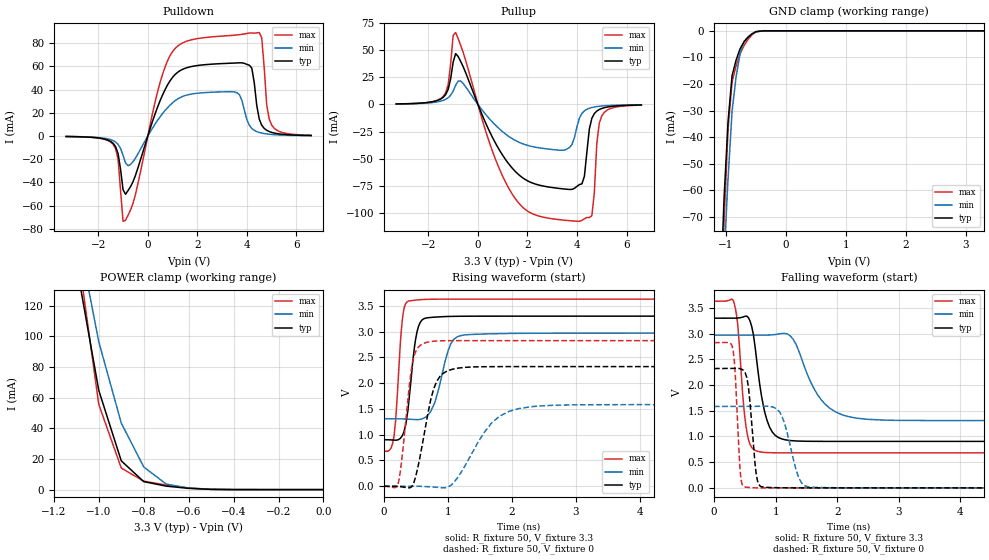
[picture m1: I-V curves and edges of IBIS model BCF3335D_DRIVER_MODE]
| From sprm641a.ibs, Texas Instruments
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|   Model Cell BCF3335D_DRIVER_MODE
|BCF3335D_DRIVER_MODE
[Model]   BCF3335D_DRIVER_MODE
Model_type   I/O
Polarity   Non-Inverting
Enable   Active-Low
Vinl =  0.8
Vinh =  2
Cref =  15.0000pF
Rref =  100.0000M
Vref =  0V
Vmeas =  1.65
C_comp   1.199917p   1.06526p   1.338254p
[Model Spec]
Vinl   0.8   0.8   0.8
Vinh   2   2   2
[Temperature Range]   25   155   -40
[Voltage Range]   3.3   2.97   3.63
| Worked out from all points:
|   slope of the pulldown table from 0 to 0.495 V, typ, clamps not added: 16.3 ohm
|   slope of the pullup table from 0 to 0.495 V, typ, clamps not added: 18.9 ohm
|   GND clamp passes 1 mA (typ) near -0.56 V on its own axis
|   POWER clamp passes 1 mA (typ) near -0.61 V on its own axis
|   rising waveform, R_fixture 50, V_fixture 3.3: 20-80 % time 127ps typ, 205ps min, 90.4ps max; typ from 0.903 V to 3.3 V
|   rising waveform, R_fixture 50, V_fixture 0: 20-80 % time 223ps typ, 490ps min, 144ps max; typ from 0 V to 2.32 V
|   falling waveform, R_fixture 50, V_fixture 3.3: 20-80 % time 186ps typ, 409ps min, 117ps max; typ from 3.3 V to 0.904 V
|   falling waveform, R_fixture 50, V_fixture 0: 20-80 % time 98.6ps typ, 200ps min, 70.6ps max; typ from 2.32 V to 0 V
| Nom Voltages:
|   VDD=1.2, VDDS=3.3, VSS=0
| Min Voltages:
|   VDD=1.08, VDDS=2.97, VSS=0
| Max Voltages:
|   VDD=1.32, VDDS=3.63, VSS=0
[POWER_clamp]
|   voltage   I(typ)   I(min)   I(max)
-3.3V     2.333A     2.602A     3.083A
-1.1V     147.4mA    172.1mA    162.2mA
-1.067V   119.9mA    146.9mA    126.6mA
-1.033V   92.31mA    121.7mA    91.13mA
-1V       64.75mA    96.51mA    55.62mA
-900mV    18.8mA     43.48mA    14.07mA
-800mV    5.216mA    14.79mA    5.52mA
-700mV    2.264mA    3.616mA    2.996mA
-600mV    818uA      964.4uA    1.072mA
-500mV    141.2uA    235.3uA    153.9uA
0V        61.19pA    4.167nA    14.54pA
[Pulldown]
|   voltage   I(typ)   I(min)   I(max)
-3.3V     -403uA     -368.2uA   -387.5uA
-1.4V     -6.274mA   -3.954mA   -7.17mA
-1V       -46.14mA   -16.63mA   -73.44mA
-900mV    -50.15mA   -23.11mA   -72.63mA
1V        50.58mA    28.66mA    72.73mA
3.5V      62.89mA    37.99mA    86.89mA
4.1V      61.02mA    9.239mA    88.75mA
4.5V      14.64mA    3.109mA    89.14mA
4.6V      9.338mA    2.567mA    84.75mA
4.8V      4.978mA    1.834mA    27.29mA
5V        3.152mA    1.372mA    9.538mA
6.6V      452.9uA    340.1uA    623.8uA
[Pullup]
|   voltage   I(typ)   I(min)   I(max)
-3.3V     473.5uA    403.7uA    428uA
-1.4V     6.607mA    3.754mA    7.428mA
-900mV    46.96mA    17.64mA    66.4mA
500mV     -26.43mA   -14.16mA   -37.58mA
1.4V      -59.24mA   -31.81mA   -83.35mA
3.5V      -78.14mA   -42.09mA   -107mA
4.1V      -74.04mA   -12.64mA   -108mA
4.3V      -66.34mA   -5.902mA   -105.5mA
4.6V      -12.82mA   -2.843mA   -102.8mA
4.8V      -6.143mA   -1.976mA   -36.29mA
5V        -3.729mA   -1.451mA   -10.6mA
6.6V      -503.1uA   -348.9uA   -638.7uA
[GND_clamp]
|   voltage   I(typ)   I(min)   I(max)
-3.3V     -1.904A    -1.594A    -3.188A
-1.1V     -103.1mA   -119.1mA   -123.9mA
-1.033V   -62.88mA   -85.18mA   -71.76mA
-966.7mV  -34.15mA   -55.59mA   -36.87mA
-900mV    -16.92mA   -30.32mA   -19.28mA
-833.3mV  -11.05mA   -17.4mA    -13.25mA
-766.7mV  -6.782mA   -8.629mA   -8.671mA
-700mV    -4.106mA   -3.992mA   -5.544mA
-566.7mV  -1.13mA    -1.152mA   -1.479mA
-500mV    -290.2uA   -424.2uA   -331.9uA
-300mV    -598.5nA   -5.196uA   -296.8nA
3.3V      61.19pA    6.786uA    8.042pA
[Ramp]
| variable   typ   min   max
dV/dt_f   1.460909/0.18806468n  1.0180177/0.41349997n  1.7939123/0.11797372n
dV/dt_r  1.4112738/0.22589037n 0.96781391/0.49582028n  1.7110268/0.14557805n
R_load = 50
[Rising Waveform]
R_fixture = 50
V_fixture = 3.3
V_fixture_min = 2.97
V_fixture_max = 3.63
|   time   V(typ)   V(min)   V(max)
0s        903.3mV    1.31V      681.1mV
157ps     893.5mV    1.31V      970.8mV
313.7ps   1.059V     1.306V     3.443V
443.7ps   2.339V     1.295V     3.604V
512.8ps   2.975V     1.292V     3.613V
611ps     3.241V     1.316V     3.623V
794ps     3.281V     1.622V     3.629V
1.047ns   3.295V     2.768V     3.63V
1.325ns   3.299V     2.942V     3.63V
20.05ns   3.3V       2.97V      3.63V
[Rising Waveform]
R_fixture = 50
V_fixture = 0
V_fixture_min = 0
V_fixture_max = 0
|   time   V(typ)   V(min)   V(max)
0s        0V         0V         0V
222ps     -4.677mV   0V         51.23mV
400.1ps   -30mV      0V         1.999V
463.7ps   58.3mV     0V         2.49V
743.4ps   1.737V     -11.96mV   2.81V
872ps     2.126V     -25.77mV   2.821V
1.074ns   2.272V     53.41mV    2.825V
1.683ns   2.32V      1.229V     2.825V
2.41ns    2.321V     1.556V     2.825V
20.01ns   2.321V     1.584V     2.825V
[Falling Waveform]
R_fixture = 50
V_fixture = 3.3
V_fixture_min = 2.97
V_fixture_max = 3.63
|   time   V(typ)   V(min)   V(max)
0s        3.3V       2.97V      3.63V
328.6ps   3.299V     2.97V      3.581V
384ps     3.303V     2.97V      3.175V
535.6ps   3.335V     2.97V      1.064V
638.2ps   2.981V     2.97V      750.4mV
781.7ps   1.71V      2.969V     693.2mV
1.096ns   952.7mV    3.001V     681mV
1.797ns   903.9mV    1.635V     681.1mV
2.48ns    903.9mV    1.334V     681.1mV
20.05ns   903.9mV    1.309V     681.1mV
[Falling Waveform]
R_fixture = 50
V_fixture = 0
V_fixture_min = 0
V_fixture_max = 0
|   time   V(typ)   V(min)   V(max)
0s        2.321V     1.584V     2.825V
292.3ps   2.323V     1.583V     2.763V
430.1ps   2.314V     1.583V     243.7mV
548ps     2.03V      1.584V     8.967mV
682.9ps   281.6mV    1.586V     0V
814.8ps   13.78mV    1.589V     0V
1.062ns   2.276mV    1.479V     0V
1.375ns   0V         196.1mV    0V
1.581ns   0V         12.93mV    0V
20.01ns   0V         0V         0V
